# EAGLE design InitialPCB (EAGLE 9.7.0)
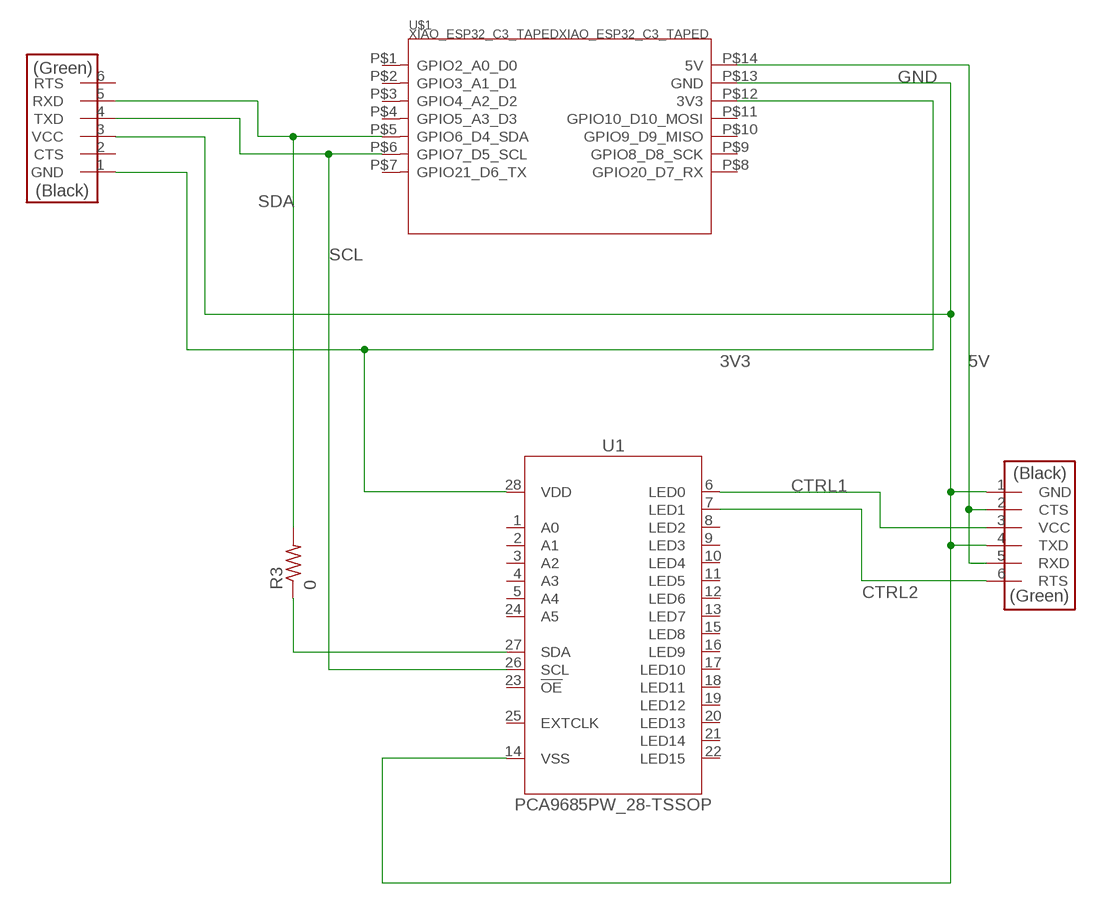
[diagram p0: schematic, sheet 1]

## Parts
R3  0  R1206  [R1206]
U1  PCA9685PW_28-TSSOP  [SOP65P640X110-28]
U$1  XIAO_ESP32_C3_TAPEDXIAO_ESP32_C3_TAPED  [XIAO_ESP32_C3_TAPED]
U$2  CONN_06_FTDI-SMD-HEADER  [1X06SMD]
U$3  CONN_06_FTDI-SMD-HEADER  [1X06SMD]

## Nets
3V3: U1.28(VDD) U$1.P$12(3V3) U$2.1(GND)
5V: U$1.P$14(5V) U$3.2(CTS) U$3.5(RXD)
CTRL1: U1.6(LED0) U$3.3(VCC)
CTRL2: U1.7(LED1) U$3.6(RTS)
GND: U1.14(VSS) U$1.P$13(GND) U$2.3(VCC) U$3.1(GND) U$3.4(TXD)
N$1: R3.1 U1.27(SDA)
SCL: U1.26(SCL) U$1.P$6(GPIO7_D5_SCL) U$2.4(TXD)
SDA: R3.2 U$1.P$5(GPIO6_D4_SDA) U$2.5(RXD)
Unconnected: U1.1(A0) U1.2(A1) U1.3(A2) U1.4(A3) U1.5(A4) U1.8(LED2) U1.9(LED3) U1.10(LED4) U1.11(LED5) U1.12(LED6) U1.13(LED7) U1.15(LED8) U1.16(LED9) U1.17(LED10) U1.18(LED11) U1.19(LED12) U1.20(LED13) U1.21(LED14) U1.22(LED15) U1.23(!OE) U1.24(A5) U1.25(EXTCLK) U$1.P$1(GPIO2_A0_D0) U$1.P$2(GPIO3_A1_D1) U$1.P$3(GPIO4_A2_D2) U$1.P$4(GPIO5_A3_D3) U$1.P$7(GPIO21_D6_TX) U$1.P$8(GPIO20_D7_RX) U$1.P$9(GPIO8_D8_SCK) U$1.P$10(GPIO9_D9_MISO) U$1.P$11(GPIO10_D10_MOSI) U$2.2(CTS) U$2.6(RTS)

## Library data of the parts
R3 = fab:R: Resistor (US Symbol)
U1 = IC_Power-Management:PCA9685PW: LED Driver IC 16 Output; CATEGORY: Power Management IC; DATASHEET: https://www.nxp.com/docs/en/data-sheet/PCA9685.pdf; DESCRIPTION: LED Driver IC 16 Output Linear PWM Dimming 25mA 28-TSSOP; INPUT_VOLTAGE: 2.3V ~ 5.5V; MANUFACTURER: NXP USA Inc.; MPN: PCA9685PW118; OPERATING_TEMPERATURE: -40°C ~ 85°C; OUTPUT_CURRENT: 25mA; OUTPUT_VOLTAGE: 5.5V; PACKAGE_SIZE: 28-TSSOP; PACKAGE_TYPE: Surface Mount; PART_STATUS: Active; ROHS: Compliant; SERIES: PCA9685; SUBCATEGORY: LED Drivers; THERMALLOSS: 0.4 W; TOPOLOGY: NA; TYPE: Linear
U$1 = fab:XIAO_ESP32_C3_TAPED
U$2 U$3 = fab:CONN_06_FTDI-SMD-HEADER

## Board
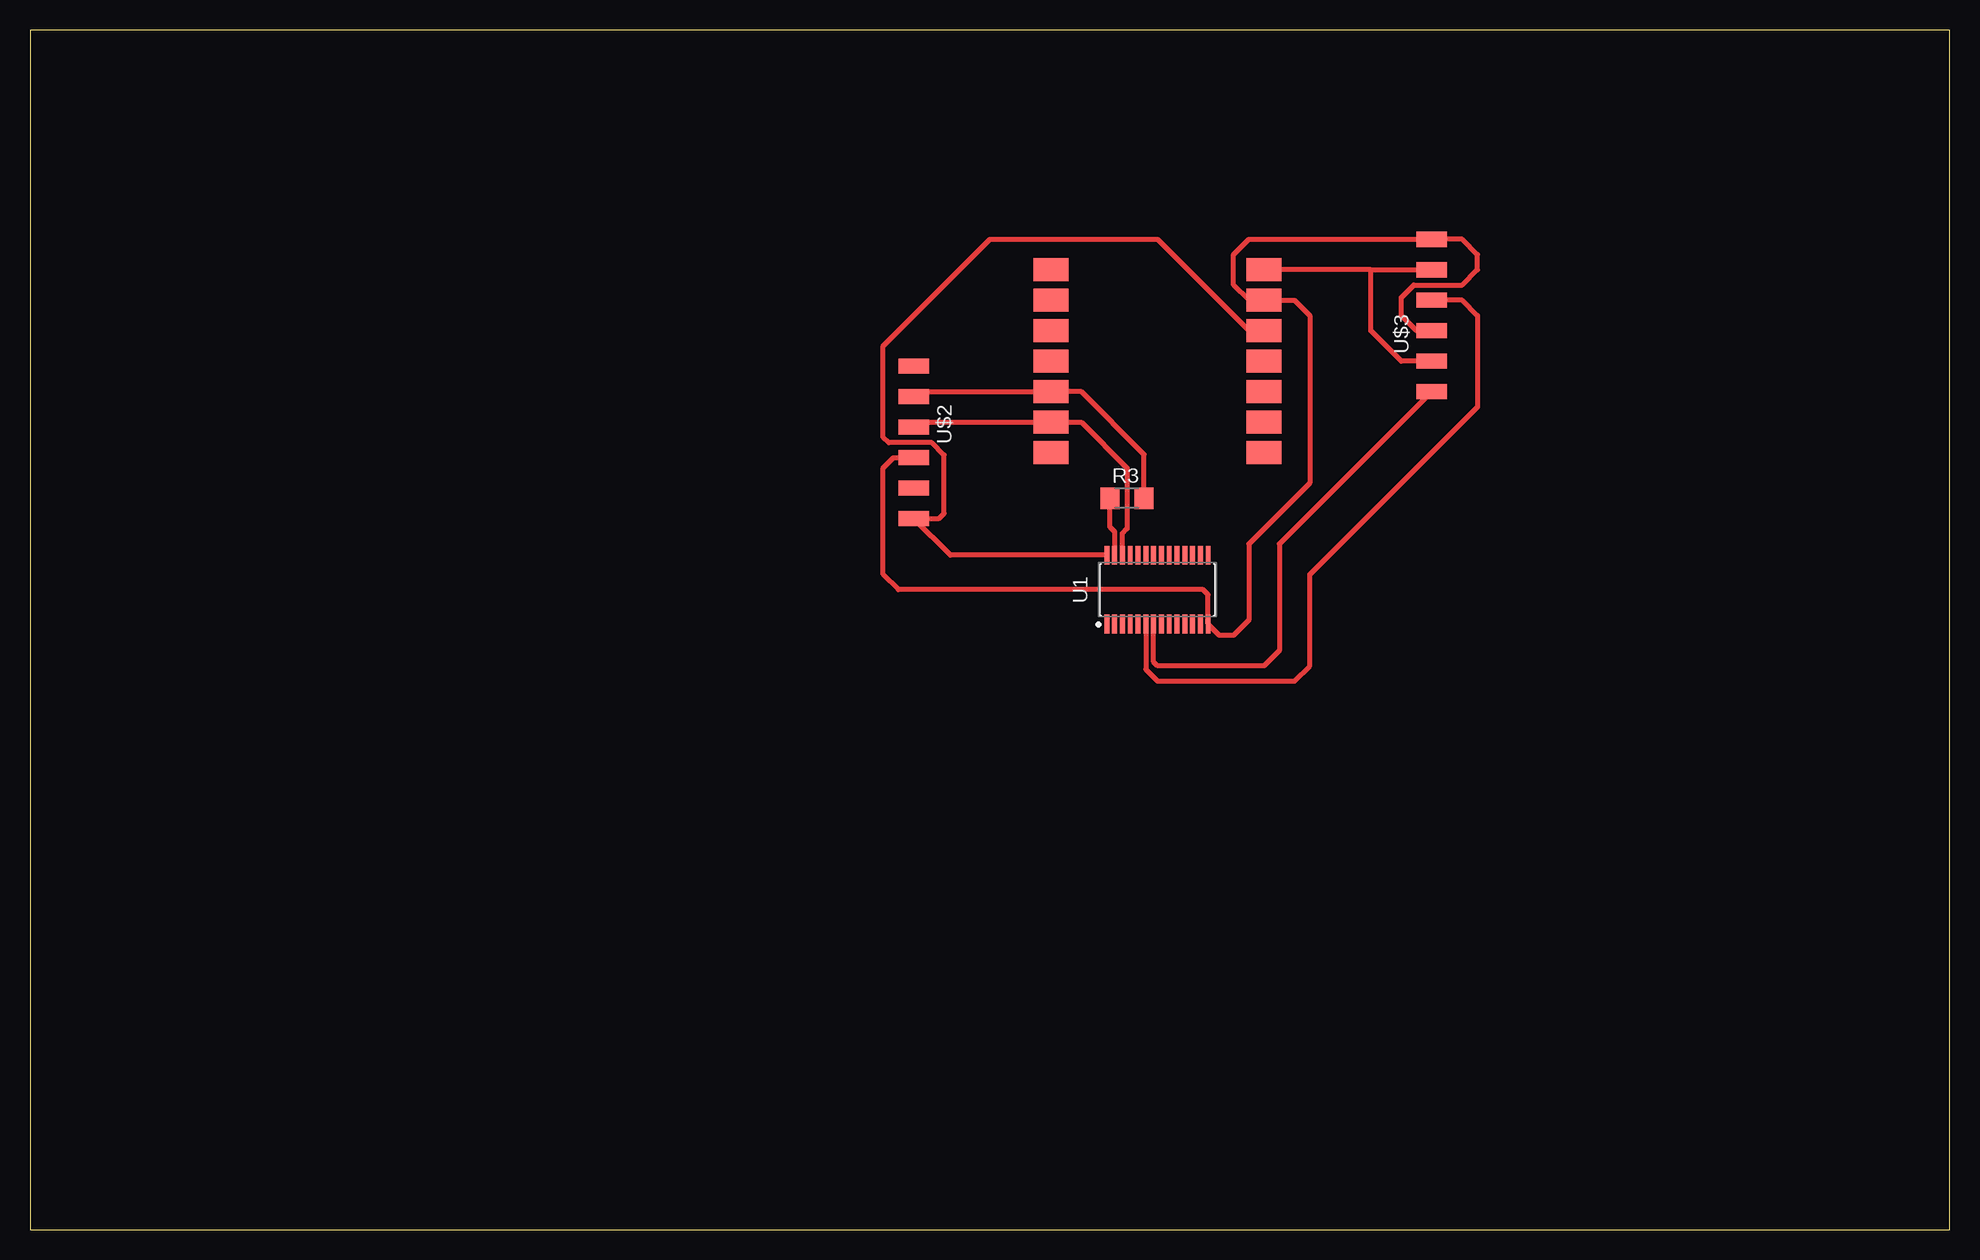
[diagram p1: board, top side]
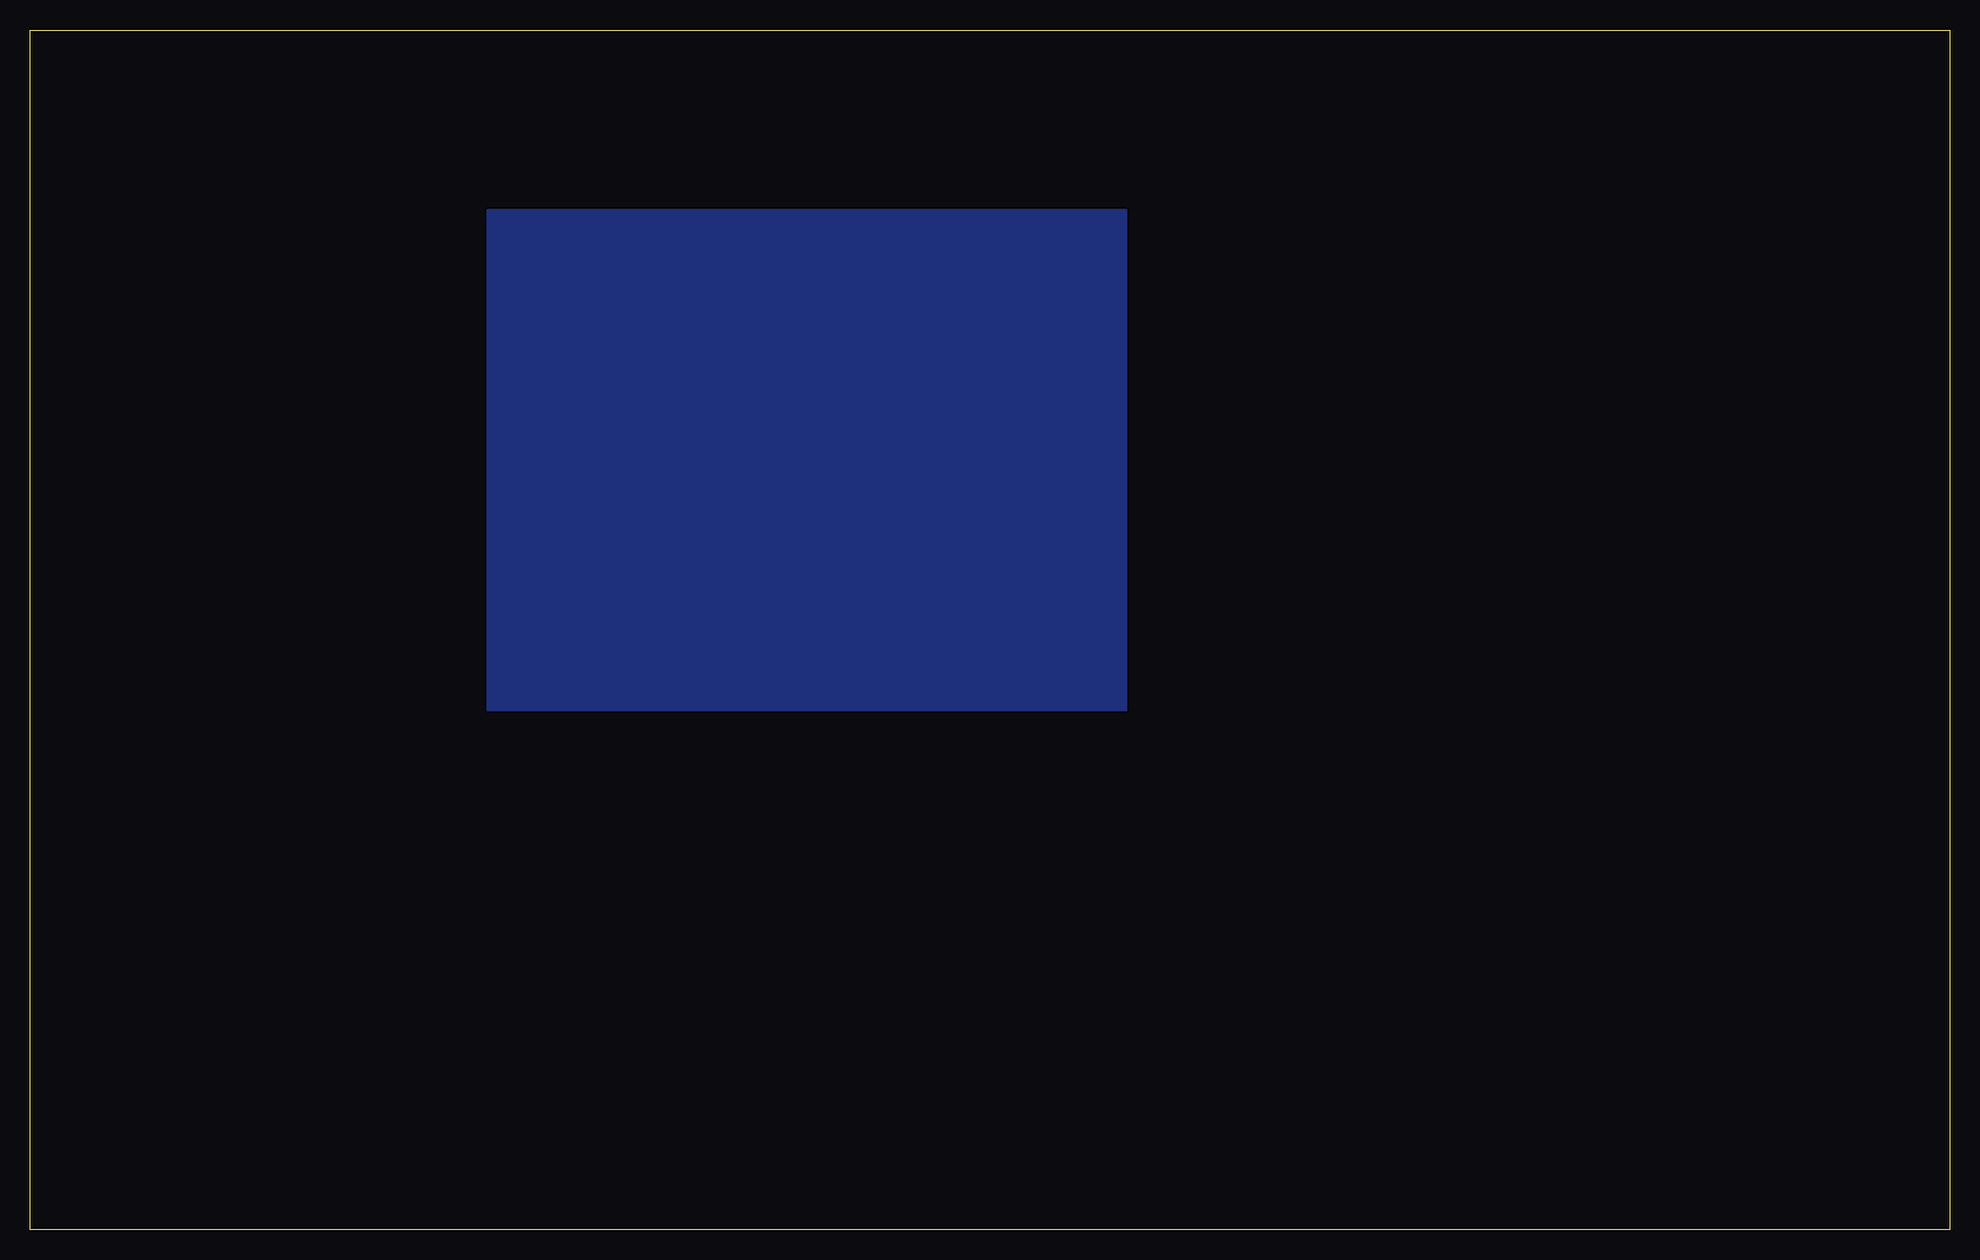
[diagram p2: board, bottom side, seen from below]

Size 160 x 100 mm. Coordinates in mm from the lower left corner, seen from the top.
Outline: 0,0 160,0 160,100 0,100 0,0
Copper layers (1*16): Top 0.035mm / dielectric 1.5mm / Bottom 0.035mm
Design rules "Fusion Electronics Design Rules": minimum track width 6mil, minimum drill 0.35mm, track to track 16mil, track to pad 16mil, pad to pad 16mil, via to via 16mil, smd to smd 6mil, copper to edge 40mil, drill to drill 6mil, minimum pad ring 10mil, minimum via ring 8mil, stop-mask expansion 4mil, vias tented up to drill 9999mil, thermal gap 10mil

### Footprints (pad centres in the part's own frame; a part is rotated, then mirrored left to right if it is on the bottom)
R1206 = smd 1.6 x 1.803: 1 -1.422,0; 2 1.422,0
SOP65P640X110-28 = smd 1.572 x 0.407: 1 -2.872,4.225; 2 -2.872,3.575; 3 -2.872,2.925; 4 -2.872,2.275; 5 -2.872,1.625; 6 -2.872,0.975; 7 -2.872,0.325; 8 -2.872,-0.325; 9 -2.872,-0.975; 10 -2.872,-1.625; 11 -2.872,-2.275; 12 -2.872,-2.925; 13 -2.872,-3.575; 14 -2.872,-4.225; 15 2.872,-4.225; 16 2.872,-3.575; 17 2.872,-2.925; 18 2.872,-2.275; 19 2.872,-1.625; 20 2.872,-0.975; 21 2.872,-0.325; 22 2.872,0.325; 23 2.872,0.975; 24 2.872,1.625; 25 2.872,2.275; 26 2.872,2.925; 27 2.872,3.575; 28 2.872,4.225
XIAO_ESP32_C3_TAPED = smd 1.905 x 2.921: P$1 0,0; P$2 -2.54,0; P$3 -5.08,0; P$4 -7.62,0; P$5 -10.16,0; P$6 -12.7,0; P$7 -15.24,0; P$8 -15.24,-17.78; P$9 -12.7,-17.78; P$10 -10.16,-17.78; P$11 -7.62,-17.78; P$12 -5.08,-17.78; P$13 -2.54,-17.78; P$14 0,-17.78
1X06SMD = smd 2.54 x 1.27: 1 0,6.35; 2 0,3.81; 3 0,1.27; 4 0,-1.27; 5 0,-3.81; 6 0,-6.35

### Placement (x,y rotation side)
R3  91.44,60.96 0 top
U1  93.98,53.34 90 top
U$1  85.09,80.01 90 top
U$2  73.66,65.62 180 top
U$3  116.84,76.2 0 top

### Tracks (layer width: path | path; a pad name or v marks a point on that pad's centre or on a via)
3V3
  Top 0.406: U1.28 76.72,56.21 U$2.1 75.78,59.27 76.2,59.69 76.2,64.58 75.18,65.6 71.56,65.6 71.12,66.04 71.12,73.66 80.01,82.55 93.98,82.55 101.6,74.93 U$1.P$12
5V
  Top 0.406: 111.76,80.01 U$3.2 | U$3.5 114.3,72.39 111.76,74.93 111.76,80.01 | 111.76,80.01 U$1.P$14
CTRL1
  Top 0.406: U1.6 93,46.7 93.98,45.72 105.41,45.72 106.68,46.99 106.68,54.61 120.65,68.58 120.65,76.2 119.38,77.47 U$3.3
CTRL2
  Top 0.406: U1.7 93.66,47.31 93.98,46.99 102.87,46.99 104.14,48.26 104.14,57.15 U$3.6
GND
  Top 0.406: U$3.4 115.57,74.93 114.3,76.2 114.3,77.7 115.34,78.74 119.38,78.74 120.65,80.01 120.65,81.28 119.38,82.55 U$3.1 101.6,82.55 100.33,81.28 100.33,78.74 101.6,77.47 U$1.P$13 105.41,77.47 106.68,76.2 106.68,62.23 101.6,57.15 101.6,50.8 100.33,49.53 99.14,49.53 U1.14 98.2,52.92 97.79,53.34 72.39,53.34 71.12,54.61 71.12,63.5 71.97,64.35 U$2.3
  pour Bottom: 68.66,43.26 121.84,43.26 121.84,85.01 68.66,85.01
N$1
  Top 0.406: U1.27 90.41,58.19 90.02,58.57 R3.1
SCL
  Top 0.406: U$2.4 74.08,67.31 U$1.P$6 87.63,67.31 91.44,63.5 91.44,58.42 91.06,58.03 U1.26
SDA
  Top 0.406: U$2.5 74.08,69.85 U$1.P$5 87.63,69.85 92.86,64.62 R3.2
